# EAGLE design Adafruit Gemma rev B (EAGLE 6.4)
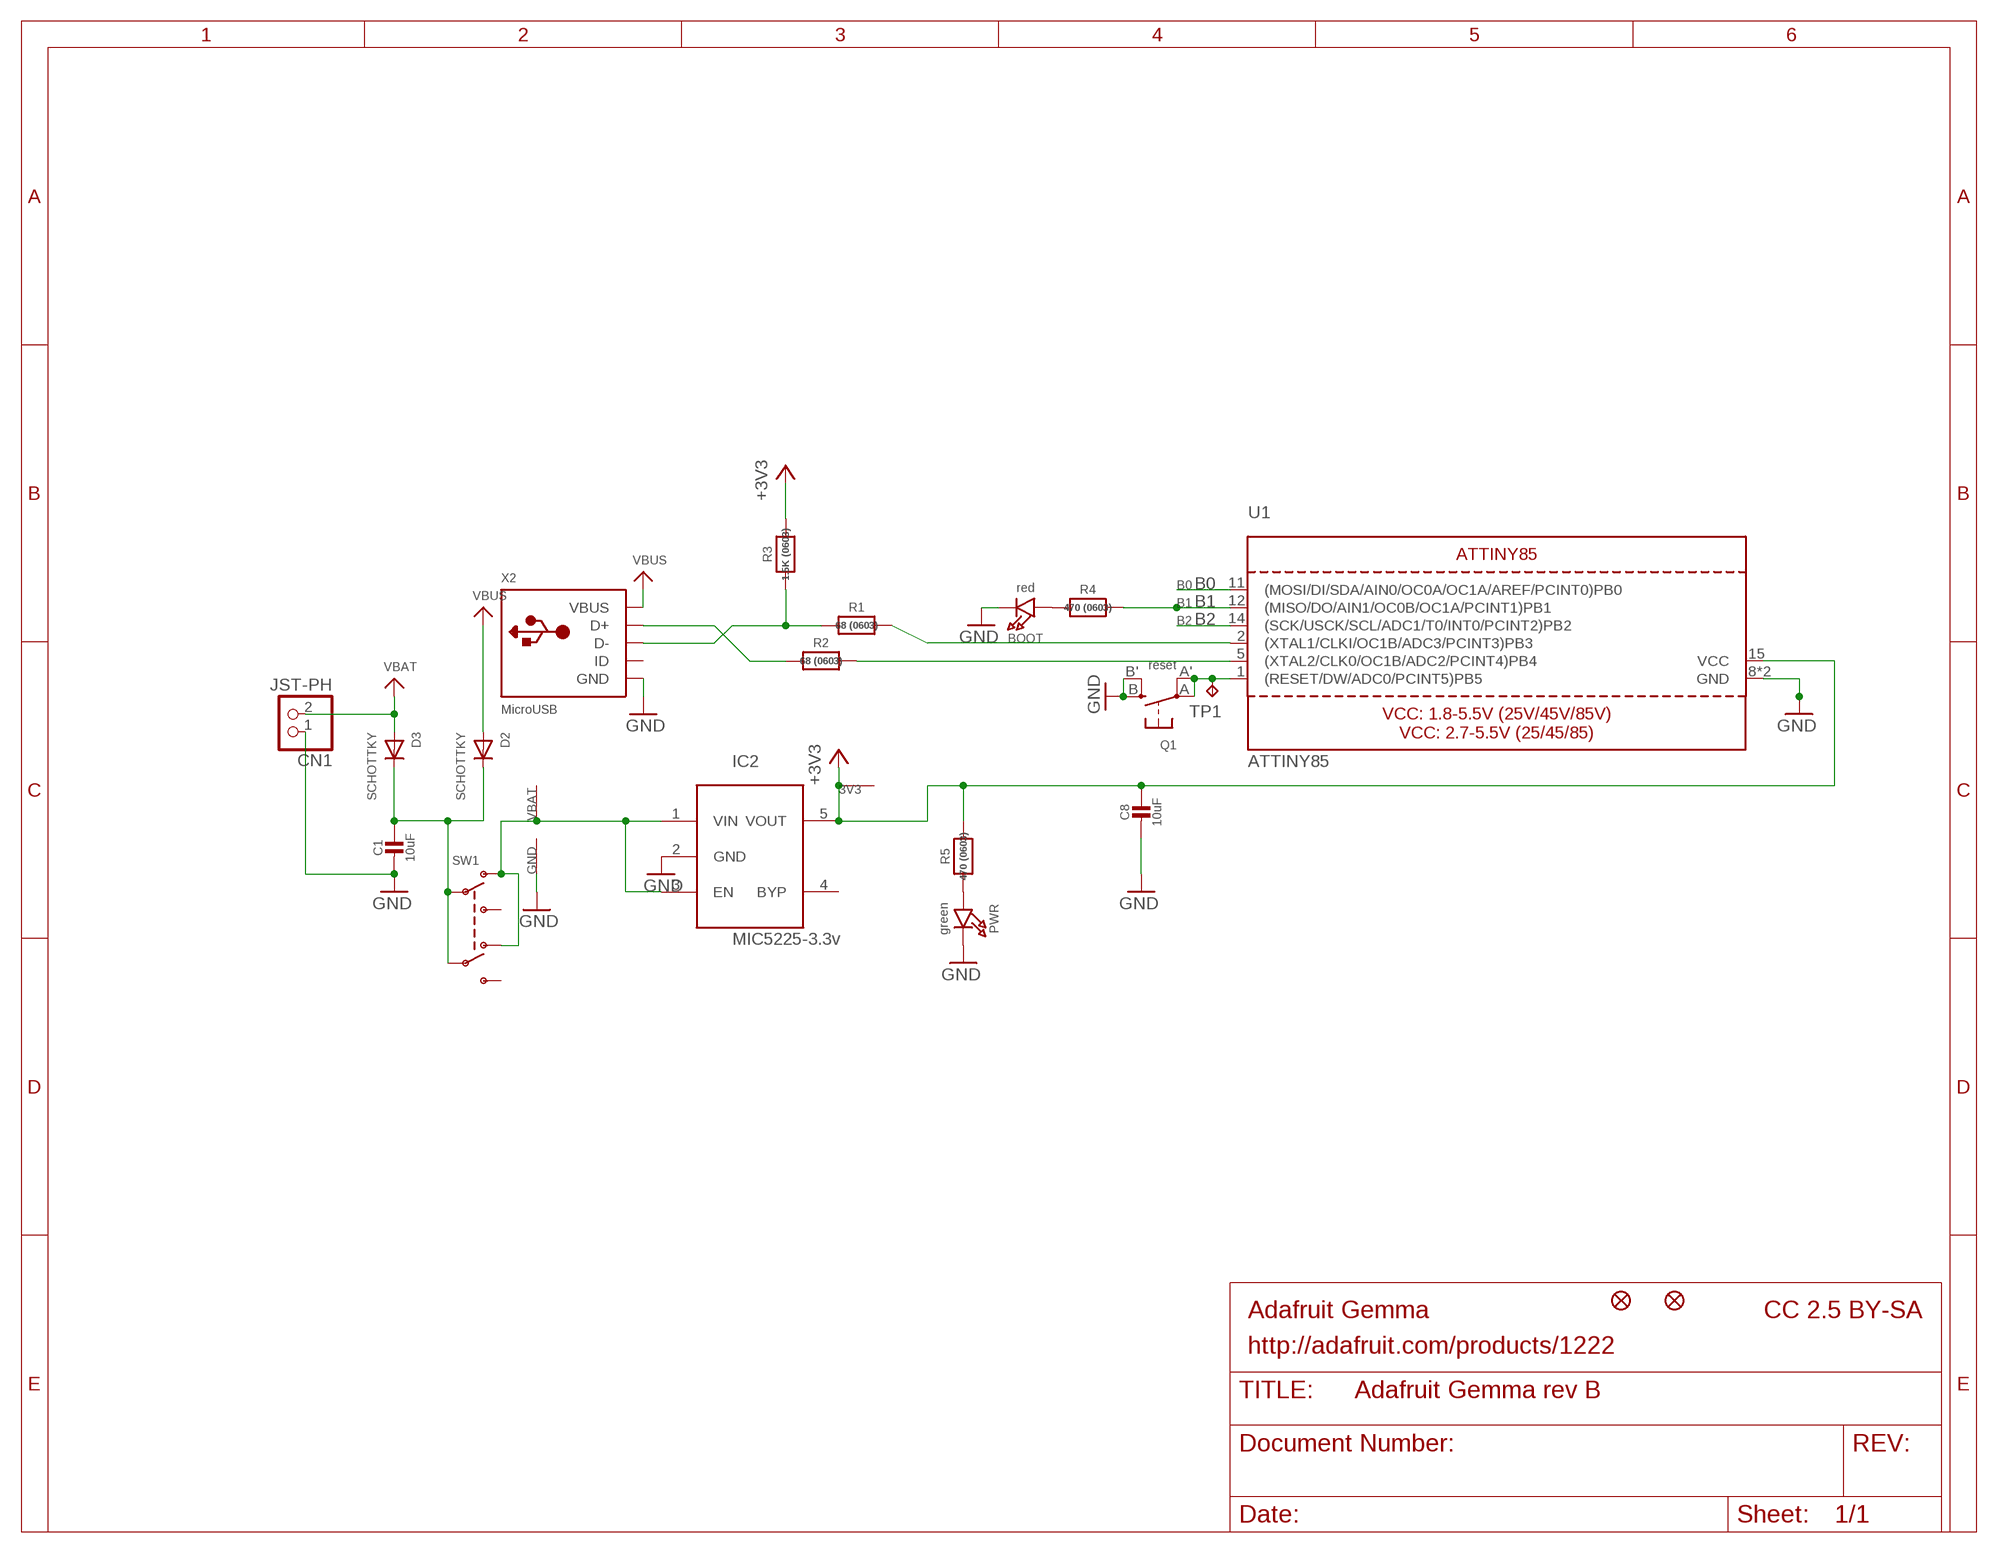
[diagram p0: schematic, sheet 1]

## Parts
3V3  SEWTAP-2.0IN  [SEWINGTAP_2.0]
B0  SEWTAP-2.0IN  [SEWINGTAP_2.0]
B1  SEWTAP-2.0IN  [SEWINGTAP_2.0]
B2  SEWTAP-2.0IN  [SEWINGTAP_2.0]
BOOT  red  LED0805_NOOUTLINE  [CHIPLED_0805_NOOUTLINE]
C1  10uF  CAP_CERAMIC0805-NOOUTLINE  [0805-NO]
C8  10uF  CAP_CERAMIC0805-NOOUTLINE  [0805-NO]
CN1  JST-PH  CON_JST_PH_2PIN  [JSTPH2]
D2  SCHOTTKY  DIODE_SOD-123FL  [SOD-123FL]
D3  SCHOTTKY  DIODE_SOD-123FL  [SOD-123FL]
GND  SEWTAP-2.0IN  [SEWINGTAP_2.0]
IC2  MIC5225-3.3v  LP298XS  [SOT23-5L]
PWR  green  LED0805_NOOUTLINE  [CHIPLED_0805_NOOUTLINE]
Q1  reset  SWITCH_TACT_SMT4.6X2.8  [BTN_KMR2_4.6X2.8]
R1  68 (0603)  RESISTOR_0603_NOOUT  [0603-NO]
R2  68 (0603)  RESISTOR_0603_NOOUT  [0603-NO]
R3  1.5K (0603)  RESISTOR_0603_NOOUT  [0603-NO]
R4  470 (0603)  RESISTOR_0603_NOOUT  [0603-NO]
R5  470 (0603)  RESISTOR_0603_NOOUT  [0603-NO]
SW1  SWITCH_DPDTEG1390  [EG1390]
TP1  TPB2,54  [B2,54]
U1  ATTINY85  [MLF20_4X4MM_0.5MM_ATMEL]
U$1  FIDUCIAL""  [FIDUCIAL_1MM]
U$6  FIDUCIAL""  [FIDUCIAL_1MM]
VBAT  SEWTAP-2.0IN  [SEWINGTAP_2.0]
X2  MicroUSB  USBMICRO_20329  [4UCONN_20329]

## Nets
+3V3: 3V3.P$1(SEW) C8.1 IC2.5(VOUT) R3.2 R5.2 U1.15(VCC)
B0: B0.P$1(SEW) U1.11((MOSI/DI/SDA/AIN0/OC0A/OC1A/AREF/PCINT0)PB0)
B1: B1.P$1(SEW) R4.2 U1.12((MISO/DO/AIN1/OC0B/OC1A/PCINT1)PB1)
B2: B2.P$1(SEW) U1.14((SCK/USCK/SCL/ADC1/T0/INT0/PCINT2)PB2)
GND: BOOT.C C1.2 C8.2 CN1.1 GND.P$1(SEW) IC2.2(GND) PWR.C Q1.B'(S1) Q1.B(S) U1.8(GND) U1.THERMAL(GND) X2.BASE@1(GND) X2.BASE@2(GND) X2.GND X2.SPRT@1(GND) X2.SPRT@2(GND) X2.SPRT@3(GND) X2.SPRT@4(GND)
N$1: Q1.A'(P1) Q1.A(P) TP1.TP U1.1((RESET/DW/ADC0/PCINT5)PB5)
N$2: R2.1 X2.D+
N$3: R1.2 U1.2((XTAL1/CLKI/OC1B/ADC3/PCINT3)PB3)
N$4: R2.2 U1.5((XTAL2/CLK0/OC1B/ADC2/PCINT4)PB4)
N$5: R1.1 R3.1 X2.D-
N$6: BOOT.A R4.1
N$7: IC2.1(VIN) IC2.3(EN) SW1.O1 SW1.O2 VBAT.P$1(SEW)
N$8: PWR.A R5.1
N$9: C1.1 D2.C D3.C SW1.P1 SW1.P2
VBAT: CN1.2 D3.A
VBUS: D2.A X2.VBUS
Unconnected: IC2.4(BYP) SW1.S1 SW1.S2 X2.ID

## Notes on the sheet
- Adafruit Gemma | CC 2.5 BY-SA
- http://adafruit.com/products/1222

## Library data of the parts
3V3 B0 B1 B2 GND VBAT = adafruit:SEWTAP
BOOT PWR = microbuilder:LED: LED
C1 C8 = microbuilder:CAP_CERAMIC: Ceramic Capacitors
CN1 = microbuilder:CON_JST_PH_2PIN: JST 2-Pin Right-Angle Connector
D2 D3 = adafruit:DIODE: Diode
IC2 = adafruit:LP298X
Q1 = microbuilder:SWITCH_TACT_SMT: SMT Tact Switches 6x6mm - Digikey: P12940SCT-ND KMR2 (4.6x2.8mm) - Digikey: 401-1426-1-ND EVQ-PQHB55 - Light Touch, 160GF (4.5x4.5mm) - Digikey: P8090SCT-ND KMT0 - KMT021 NGJ LHS (etc.) IP68/Waterproof - Digikey: CKN10289CT-ND
R1-R5 = microbuilder:RESISTOR: Resistors
SW1 = microbuilder:SWITCH_DPDT: Switch - DPDT A DPDT Switch acts like an SPDT switch, but has a pair of switches instead of just one. Vertical - 0.3A @ 6V SMT - Digikey: JS202011SCQN
TP1 = testpad:TP: Test pad
U1 = microbuilder:ATTINY85: ATTINT85
U$1 U$6 = microbuilder:FIDUCIAL: Fiducial Alignment Points; BOM: EXCLUDE
X2 = microbuilder:USB: USB Connectors USBMINIB - Surface Mount Female Mini-B USB Connector 4UConnector: 06564

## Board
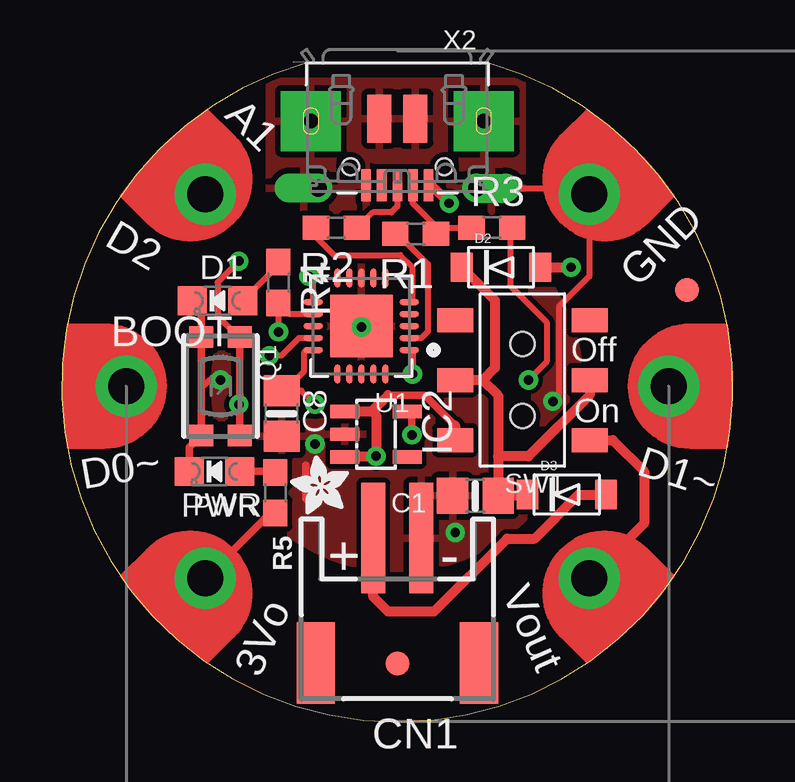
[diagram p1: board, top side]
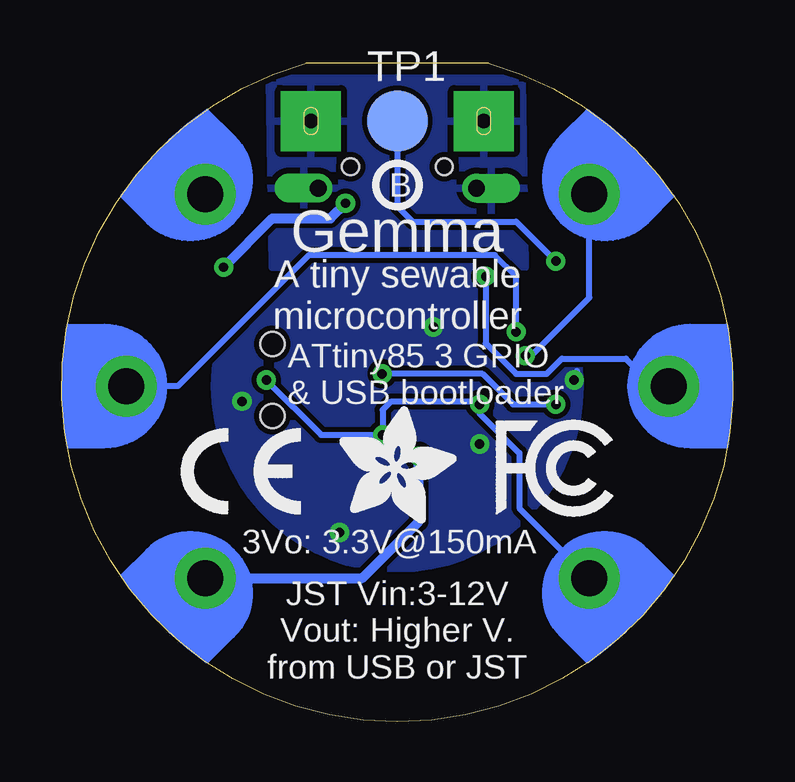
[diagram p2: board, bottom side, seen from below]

Size 27.97 x 27.46 mm. Coordinates in mm from the lower left corner, seen from the top.
Outline: 10.17,27.46 17.79,27.46 arc-328 10.17,27.46
Copper layers (1*16): Top 0.035mm / dielectric 1.5mm / Bottom 0.035mm
Design rules "adafruit *": minimum track width 8mil, minimum drill 15.5mil, track to track 8mil, track to pad 8mil, pad to pad 8mil, via to via 8mil, smd to smd 8mil, copper to edge 10mil, drill to drill 8mil, minimum pad ring 10mil, minimum via ring 8mil, stop-mask expansion 2mil, vias tented up to drill 20mil, thermal gap 10mil

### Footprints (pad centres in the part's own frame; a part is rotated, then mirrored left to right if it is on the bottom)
SEWINGTAP_2.0 = drill 1.5 pad 2.54: P$1 0,0
CHIPLED_0805_NOOUTLINE = smd 1.2 x 1.2: A 0,-1.05; C 0,1.05
0805-NO = smd 1.3 x 1.5: 1 -0.95,0; 2 0.95,0
JSTPH2 = smd 1 x 4.6: 1 -1,-3.7; 2 1,-3.7 | smd 1.6 x 3.4: NC1 -3.4,1.5; NC2 3.4,1.5
SOD-123FL = smd 0.91 x 1.22: A 1.637,0; C -1.637,0
SOT23-5L = smd 0.55 x 1.2: 1 -0.95,-1.3; 2 0,-1.3; 3 0.95,-1.3; 4 0.95,1.3; 5 -0.95,1.3
BTN_KMR2_4.6X2.8 = smd 0.9 x 1: A 2.05,0.8; A' -2.05,0.8; B 2.05,-0.8; B' -2.05,-0.8
0603-NO = smd 1.1 x 1: 1 -0.85,0; 2 0.85,0
EG1390 = smd 1 x 1.5: O1 -2.5,2.8; O2 -2.5,-2.8; P1 0,2.8; P2 0,-2.8; S1 2.5,2.8; S2 2.5,-2.8 | hole 1: 1.5,0; -1.5,0
B2,54 = smd 2.54 x 2.54: TP 0,0
MLF20_4X4MM_0.5MM_ATMEL = smd 0.8 x 0.25: 1 -2,1; 2 -2,0.5; 3 -2,0; 4 -2,-0.5; 5 -2,-1; 11 2,-1; 12 2,-0.5; 13 2,0; 14 2,0.5; 15 2,1 | smd 0.25 x 0.8: 6 -1,-2; 7 -0.5,-2; 8 0,-2; 9 0.5,-2; 10 1,-2; 16 1,2; 17 0.5,2; 18 0,2; 19 -0.5,2; 20 -1,2 | smd 2.6 x 2.6: THERMAL 0,0
FIDUCIAL_1MM = smd 1 x 1: 1 0,0
4UCONN_20329 = smd 1 x 2: BASE@1 -0.75,-2; BASE@2 0.75,-2 | smd 0.4 x 1.35: D+ 0,0.775; D- -0.65,0.775; GND 1.3,0.775; ID 0.65,0.775; VBUS -1.3,0.775 | drill 0.7 offset: SPRT@1 -3.3,0.9; SPRT@2 3.3,0.9 | drill 0.6 pad 2.5 square: SPRT@3 -3.6,-1.9; SPRT@4 3.6,-1.9 | hole 0.7: -1.95,0; 1.95,0

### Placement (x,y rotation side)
3V3  5.98,5.99 135 top
B0  2.68,14 90 top
B1  25.29,14 270 top
B2  5.98,22 45 top
BOOT  6.49,17.55 90 top
C1  17.23,9.42 180 top
C8  9.16,12.85 270 top
CN1  13.98,3.96 180 top
D2  18.3,18.95 0 top
D3  21.04,9.48 0 top
GND  21.99,22 315 top
IC2  13.1,11.99 270 top
PWR  6.36,10.44 90 top
Q1  6.62,14 270 top
R1  14.75,20.35 180 top
R2  11.44,20.6 180 top
R3  17.92,20.6 0 top
R4  9.03,18.31 270 top
R5  8.9,9.55 270 top
SW1  19.19,14.25 90 top
TP1  13.98,25.04 0 bottom
U1  12.48,16.5 180 top
U$1  26.06,17.99 90 top
U$2  [ADAFRUIT_2.5MM]  11.95,8.66 90 top
U$6  13.98,2.44 0 top
U$7  [ADAFRUIT_5MM]  16.4,8.28 0 bottom
U$8  [SYMBOL_FCC_5MM]  9.92,8.53 0 bottom
U$9  [SYMBOL_CE_5MM]  23,8.66 0 bottom
U$10  [PCBFEAT-REV-040]  13.98,22.38 0 bottom
VBAT  21.99,5.99 225 top
X2  13.98,23.14 180 top

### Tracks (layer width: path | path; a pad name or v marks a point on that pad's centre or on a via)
+3V3  (via drill 0.39)
  Top 0.254: R3.2 18.68,20.51 18.68,18.19 20.21,16.66 20.21,15.01 v19.45,14.25 | U1.15 10.18,15.5 10.08,15.4 10.08,14.6 9.29,13.8 C8.1 9.99,13.8 v10.56,13.23
  Top 0.305: R5.2 8.69,8.7 3V3.P$1 | IC2.5 14.59,12.74 v14.59,11.96
  Bottom 0.254: 3V3.P$1 8.9,8.92 8.9,11.2 10.56,12.85 v10.56,13.23 10.68,13.36 14.24,13.36 14.59,13 v14.59,11.96 17.16,11.96 v19.45,14.25
B0  (via drill 0.39)
  Top 0.254: U1.11 10.48,18.38 v10.3,18.57
  Bottom 0.254: v10.3,18.57 10.3,15.77 9.03,14.5 7.76,14.5 7.13,15.14 4.46,15.14 3.32,14 B0.P$1
B1  (via drill 0.39)
  Top 0.254: v9.03,16.25 R4.2 9.5,17 U1.12
  Bottom 0.254: v9.03,16.25 9.03,18.57 9.92,19.46 17.67,19.46 23.13,14 B1.P$1
B2  (via drill 0.39)
  Top 0.254: U1.14 9.88,16 9.15,15.27 v8.65,15.27
  Bottom 0.254: B2.P$1 5.98,17.68 8.4,15.27 v8.65,15.27 8.52,15.27
GND  (via drill 0.39)
  Top 0.254: 15.25,8.28 14.98,8.01 CN1.1 | 5.82,13.91 6.15,14.25 v6.62,14.25 | X2.SPRT@1 21.99,22.24 GND.P$1 21.99,18.57 20.72,17.3 20.72,13.61 v20.46,13.36
  Top 0.305: PWR.C 5.31,11.44 Q1.B 5.82,13.91 Q1.B' 5.82,17.17 BOOT.C | C8.2 9.35,11.9 | 10.17,10.69 10.17,9.3
  Bottom 0.254: v6.62,14.25 6.49,14.38 6.49,14.63
  other vias: 10.56,11.58 16.4,7.9 12.49,16.45
  pour Bottom: 6.36,14 arc90 13.98,6.38 arc90 21.6,14 arc90 13.98,21.62 arc90
  pour Bottom: 8.78,26.82 8.65,18.95 19.19,18.95 19.32,26.82
  pour Top: 6.36,14 arc90 13.98,6.38 arc90 21.6,14 arc90 13.98,21.62 arc90
  pour Top: 8.65,26.7 8.65,18.95 19.19,18.95 19.19,26.7
N$1  (via drill 0.39)
  Top 0.254: 7.51,13.36 v7.38,13.23 7.42,13.2 Q1.A | v7.38,19.2 6.49,18.31 6.49,16.92 7.36,16.05 Q1.A' | U1.1 14.6,15.5 14.62,15.47 v14.62,14.5
  Top 0.305: Q1.A Q1.A'
  Bottom 0.254: v7.38,13.23 9.16,13.23 10.43,14.5 v14.62,14.5 | TP1.TP 13.98,21.49 13.35,20.85 9.03,20.85 v7.38,19.2
N$2
  Top 0.254: X2.D+ 13.98,21.49 13.73,21.23 12.97,21.23 12.33,20.6 R2.1
N$3
  Top 0.254: U1.2 14.98,16 15.25,16.27 15.25,19.08 13.98,20.35 R1.2
N$4
  Top 0.254: U1.5 14.62,17.63 14.62,18.95 14.11,19.46 11.36,19.46 10.59,20.22 R2.2
N$5
  Top 0.254: 15.85,20.38 15.76,20.47 | 15.76,20.47 14.62,21.62 14.62,22.35 X2.D- | R1.1 15.76,20.51 | R3.1 15.85,20.6 15.76,20.51 | 15.76,20.51 15.76,20.47
N$6
  Top 0.254: R4.1 8.99,19.16 8.99,19 BOOT.A
N$7  (via drill 0.39)
  Top 0.305: 13.6,13.61 15.13,13.61 16.39,12.35
  Top 0.406: SW1.O2 22.96,11.75 24.27,10.44 24.27,8.28 VBAT.P$1 | IC2.1 12.93,12.94 | 12.93,12.94 13.6,13.61 | 16.39,12.35 SW1.O1 | IC2.3 11.83,11.07 v13.1,11.07 13.1,12.77 12.93,12.94
  Bottom 0.406: VBAT.P$1 15.45,5.99 13.1,8.35 v13.1,11.07
N$8
  Top 0.305: PWR.A 8.87,10.44 R5.1
N$9
  Top 0.254: D3.C 19.35,9.42
  Top 0.406: D2.C 18.05,17.57 18.05,14.76 17.54,14.25 | 17.54,14.25 18.18,13.61 18.18,11.07 | 17.54,14.25 SW1.P1 | SW1.P2 21.99,13.62 19.44,11.07 18.18,11.07 | 18.18,11.07 C1.1 19.35,9.42
VBAT
  Top 0.406: CN1.2 12.98,5.22 13.6,4.6 15.51,4.6 18.56,7.65 19.7,7.65 21.53,9.48 D3.A
VBUS  (via drill 0.39)
  Top 0.406: X2.VBUS 15.39,22.36 v16.14,21.62 | D2.A v21.22,18.95
  Bottom 0.406: v16.14,21.62 16.78,20.98 19.19,20.98 v21.22,18.95

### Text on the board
tPlace: A1 | D2 | D1 | GND | Off | On | D0~ | D1~ | PWR | + | - | Vout | 3Vo
bPlace: Gemma | A tiny sewable / microcontroller | ATtiny85 3 GPIO | & USB bootloader | 3Vo: 3.3V@150mA | JST Vin:3-12V / Vout: Higher V. / from USB or JST
tDocu: SCL/SCK | GND | SDA/MOSI | MISO | 3-16VDC

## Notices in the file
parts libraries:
microbuilder: This work is placed in the public domain, and may be freely used for commercial and non-commercial work with the following conditions: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
